ORGANIZATION_BLOCK MAIN:OB1
TITLE=

BEGIN
NETWORK 1
LD I0.6
= S0.0

NETWORK 2
LDN I0.6
= S0.1

NETWORK 3
LSCR S0.0

NETWORK 4
LD I1.4
O M2.1
A I0.2
A I0.7
A I1.3
= M2.1

NETWORK 5
LD M2.1
A I0.0
= M0.1

NETWORK 6
LD M2.1
A I0.1
A I0.5
= M0.0

NETWORK 7
SCRE

NETWORK 8
LSCR S0.1

NETWORK 9
LD I1.0
A I0.0
= M1.1

NETWORK 10
LD I0.1
A I0.5
AN M2.0
A I1.2
= M1.0

NETWORK 11
SCRE

NETWORK 12
LD I1.1
= Q0.2

NETWORK 13
LD M0.0
O M1.0
= Q0.1

NETWORK 14
LD M0.1
O M1.1
= Q0.0

NETWORK 15
LD Q0.1
= Q0.3

NETWORK 16
LDN I0.2
= Q0.4

NETWORK 17
LDN I0.1
= Q0.5

NETWORK 18
LD I0.6
= Q0.6

NETWORK 19
LDN I0.2
S M2.0 1

NETWORK 20
LD I0.2
AN I1.2
EU
R M2.0 1

END_ORGANIZATION_BLOCK

